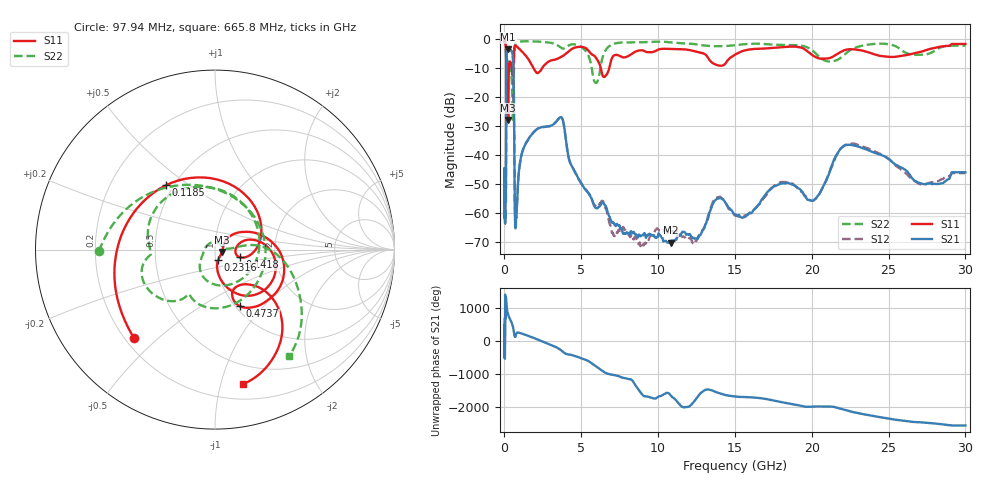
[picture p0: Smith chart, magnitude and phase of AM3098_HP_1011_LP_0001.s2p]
! Date/Time: Thu, Feb 28, 2019 8:42 AM
! Network Analyzer: Agilent Technologies E8364B Rev: A.07.50.67
! Sweep from 0.010 to 30.000 GHz, 1601 Points, Sweep Type: LOG
! Power Supply: 5.023 V, 0.002 A
# Hz S DB R 50
!freq MagS11 AngS11 MagS21 AngS21 MagS12 AngS12 MagS22 AngS22
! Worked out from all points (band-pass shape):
!   1601 points, 10 MHz to 30 GHz, reference 50 ohm
!   highest |S21| = -3.36 dB at 241.1 MHz (marker M1); lowest = -70.2 dB at 10.81 GHz (marker M2)
!   |S21| within 3 dB of the highest: 136.6 MHz to 551.6 MHz (415 MHz wide, 121 % of centre)
!   lowest |S11| = -27.8 dB at 239.9 MHz (marker M3), VSWR 1.09, Z = 54 - j1.49 ohm
!   |S11| at or under -10 dB: 200.1 MHz to 293.7 MHz (93.67 MHz wide, 37.9 % of centre); 1.898 GHz to 2.44 GHz (542 MHz wide, 25 % of centre); 6.274 GHz to 6.817 GHz (542.2 MHz wide, 8.28 % of centre)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
!   |S22| runs from -27.7 to -0.5 dB; largest |S21 - S12| = 0.0095
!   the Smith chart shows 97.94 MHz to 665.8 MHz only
!   S11 on the Smith chart (normalised r, x): 97.94 MHz: 0.24, -0.42; 118.5 MHz: 0.45, +0.41; 141.8 MHz: 1.32, -0.11; 231.6 MHz: 1.03, -0.12; 473.7 MHz: 1.05, -0.75; 665.8 MHz: 0.33, -1.18
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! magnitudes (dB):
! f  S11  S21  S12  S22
! 10 MHz  -0.3  -44.5  -45.8  -0.5
! 38.04 MHz  -0.4  -59.7  -58.8  -0.7
! 97.94 MHz  -3.5  -51.8  -51.3  -3.8
! 118.5 MHz  -6.9  -19.8  -19.8  -10.8
! 141.8 MHz  -16.8  -5.4  -5.4  -10.8
! 144.7 MHz  -18.2  -5.1  -5.1  -10.8
! 190.6 MHz  -9.0  -3.9  -3.9  -7.2
! 231.6 MHz  -24.5  -3.4  -3.4  -8.9
! 239.9 MHz  -27.8  -3.4  -3.3  -9.0
! 241.1 MHz  -27.7  -3.4  -3.3  -8.9
! 473.7 MHz  -9.3  -4.1  -4.1  -13.9
! 550.5 MHz  -11.9  -6.3  -6.3  -27.4
! 605.4 MHz  -5.6  -15.6  -15.6  -11.6
! 665.8 MHz  -2.3  -53.8  -53.6  -2.8
! 724.9 MHz  -2.1  -65.0  -63.0  -1.4
! 2.084 GHz  -11.5  -31.1  -31.0  -0.7
! 3.704 GHz  -6.0  -26.8  -26.8  -2.9
! 7.926 GHz  -6.0  -67.0  -66.2  -1.0
! 10.81 GHz  -3.2  -70.2  -66.8  -1.0
! 20.1 GHz  -5.6  -55.6  -55.6  -4.1
! 22.56 GHz  -3.4  -36.4  -36.0  -3.5
! 30 GHz  -1.6  -45.8  -46.1  -2.1
